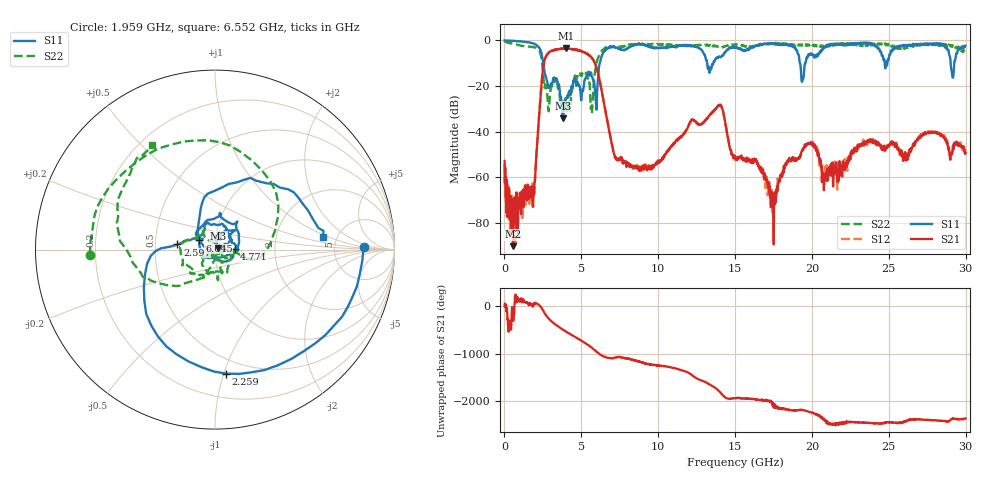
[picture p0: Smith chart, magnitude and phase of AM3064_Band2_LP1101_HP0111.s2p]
# Hz S DB R 50.0
!freq dBS11 angS11 dBS21 angS21 dBS12 angS12 dBS22 angS22
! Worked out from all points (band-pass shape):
!   1600 points, 10 MHz to 29.98 GHz, reference 50 ohm
!   highest |S21| = -3.52 dB at 4.002 GHz (marker M1); lowest = -90.2 dB at 553.6 MHz (marker M2)
!   |S21| within 3 dB of the highest: 2.744 GHz to 5.495 GHz (2.752 GHz wide, 66.8 % of centre); 5.517135 GHz to 5.52261 GHz (5.474 MHz wide, 0.0992 % of centre)
!   lowest |S11| = -34.2 dB at 3.796 GHz (marker M3), VSWR 1.04, Z = 51.9 + j0.67 ohm
!   |S11| at or under -10 dB: 2.53 GHz to 6.199 GHz (3.669 GHz wide, 84.1 % of centre); 13.18 GHz to 13.58 GHz (396.7 MHz wide, 2.96 % of centre); 19.23 GHz to 19.58 GHz (355 MHz wide, 1.83 % of centre)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
!   |S22| runs from -34.1 to -0.2 dB; largest |S21 - S12| = 0.021
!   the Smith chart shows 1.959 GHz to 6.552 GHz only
!   S11 on the Smith chart (normalised r, x): 1.959 GHz: 11, +1; 2.259 GHz: 0.38, -1.02; 2.597 GHz: 0.65, +0.04; 4.771 GHz: 1.25, +0.01; 6.045 GHz: 0.84, +0.09; 6.552 GHz: 3.88, +0.85
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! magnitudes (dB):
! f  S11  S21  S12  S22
! 10 MHz  0.0  -52.8  -54.3  -0.2
! 553.6 MHz  -0.2  -90.2  -69.0  -1.4
! 1.959 GHz  -1.6  -62.2  -64.5  -3.1
! 2.259 GHz  -3.2  -32.6  -32.6  -4.4
! 2.597 GHz  -13.5  -9.0  -9.0  -20.7
! 3.796 GHz  -34.2  -3.6  -3.6  -30.9
! 4.002 GHz  -25.3  -3.5  -3.6  -27.8
! 4.771 GHz  -19.2  -4.4  -4.1  -16.2
! 5.015 GHz  -24.5  -4.8  -4.7  -15.5
! 5.671 GHz  -15.6  -7.7  -7.5  -30.3
! 6.045 GHz  -20.0  -13.2  -13.1  -8.5
! 6.552 GHz  -4.3  -30.3  -30.4  -3.3
! 7.32 GHz  -3.1  -52.2  -51.6  -2.6
! 10 GHz  -3.4  -53.4  -53.5  -1.8
! 13.97 GHz  -7.0  -28.5  -28.3  -2.7
! 15 GHz  -3.0  -51.5  -52.5  -1.9
! 17.46 GHz  -1.3  -69.9  -68.4  -1.4
! 19.37 GHz  -17.9  -48.2  -48.1  -2.1
! 19.99 GHz  -5.9  -45.3  -45.2  -1.8
! 20.8 GHz  -2.8  -58.8  -63.1  -2.5
! 25 GHz  -8.0  -46.6  -46.1  -1.7
! 29.98 GHz  -2.3  -49.3  -48.3  -4.6
